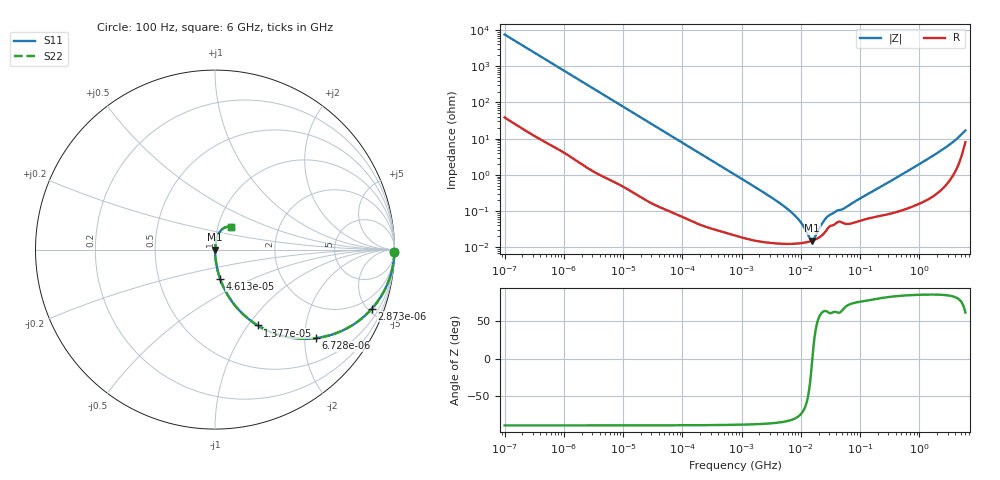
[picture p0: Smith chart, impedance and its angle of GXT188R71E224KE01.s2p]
!Murata Part Number: GXT188R71E224KE01
!These Parameters are Measured in Series Mode Connection
!Data Generated on Jan 08, 2026
!  o--ll--o
!Port1  Port2
!  o------o
!Operation Temp=25[degC], DC Bias Voltage=0[V]
!Freq. Start=100[Hz] Stop=6[GHz] 401[Steps]
# Hz S RI R 50
!Freq.(Hz) S11(Real) S11(Imag) S21(Real) S21(Imag) S12(Real) S12(Imag) S22(Real) S22(Imag)
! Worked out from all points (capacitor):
!   401 points, 100 Hz to 6 GHz, reference 50 ohm
!   read as one part in series: C = 211 nF near 109 Hz
!   lowest |Z| = 15.2 mohm at 15.56 MHz (marker M1)
!   series resonance near 15.68 MHz, so ESL is about 490 pH
!   S11 on the Smith chart (normalised r, x): 100 Hz: open; 2.873 kHz: 1.03, -5.30; 6.728 kHz: 1.01, -2.27; 13.77 kHz: 1.01, -1.11; 46.13 kHz: 1.00, -0.33; 6 GHz: 1.16, +0.30
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100  0.9998 -0.0133  0.000244 0.0133  0.000244 0.0133  0.9998 -0.0133
600  0.9934 -0.0786  0.00663 0.0786  0.00663 0.0786  0.9934 -0.0786
2008  0.9337 -0.2462  0.0663 0.2462  0.0663 0.2462  0.9337 -0.2462
2873  0.8741 -0.3292  0.1259 0.3292  0.1259 0.3292  0.8741 -0.3292
6728  0.5625 -0.4932  0.4375 0.4932  0.4375 0.4932  0.5625 -0.4932
13772  0.2375 -0.4225  0.7625 0.4225  0.7625 0.4225  0.2375 -0.4225
22537  0.1053 -0.3039  0.8947 0.3039  0.8947 0.3039  0.1053 -0.3039
40335  0.0362 -0.1834  0.9638 0.1834  0.9638 0.1834  0.0362 -0.1834
46134  0.0281 -0.1618  0.9719 0.1618  0.9719 0.1618  0.0281 -0.1618
141303  0.00351 -0.0545  0.9965 0.0545  0.9965 0.0545  0.00351 -0.0545
774597  0.000312 -0.01  0.9997 0.01  0.9997 0.01  0.000312 -0.01
3103719  0.000138 -0.00244  0.9999 0.00244  0.9999 0.00244  0.000138 -0.00244
6353432  0.000125 -0.00104  0.9999 0.00104  0.9999 0.00104  0.000125 -0.00104
9506416  0.000128 -0.000528  0.9999 0.000528  0.9999 0.000528  0.000128 -0.000528
1.422411e7  0.000145 -9.89e-05  0.9999 9.89e-05  0.9999 9.89e-05  0.000145 -9.89e-05
1.555665e7  0.000152 -7.6e-06  0.9998 7.6e-06  0.9998 7.6e-06  0.000152 -7.6e-06
1.701401e7  0.00016 8.41e-05  0.9998 -8.41e-05  0.9998 -8.41e-05  0.00016 8.41e-05
2.327686e7  0.000221 0.00042  0.9998 -0.00042  0.9998 -0.00042  0.000221 0.00042
2.911731e7  0.000347 0.000649  0.9997 -0.000649  0.9997 -0.000649  0.000347 0.000649
3.124326e8  0.000873 0.00635  0.9991 -0.00635  0.9991 -0.00635  0.000873 0.00635
2.240541e9  0.00554 0.0445  0.9945 -0.0445  0.9945 -0.0445  0.00554 0.0445
6e9  0.0911 0.1246  0.9089 -0.1246  0.9089 -0.1246  0.0911 0.1246
